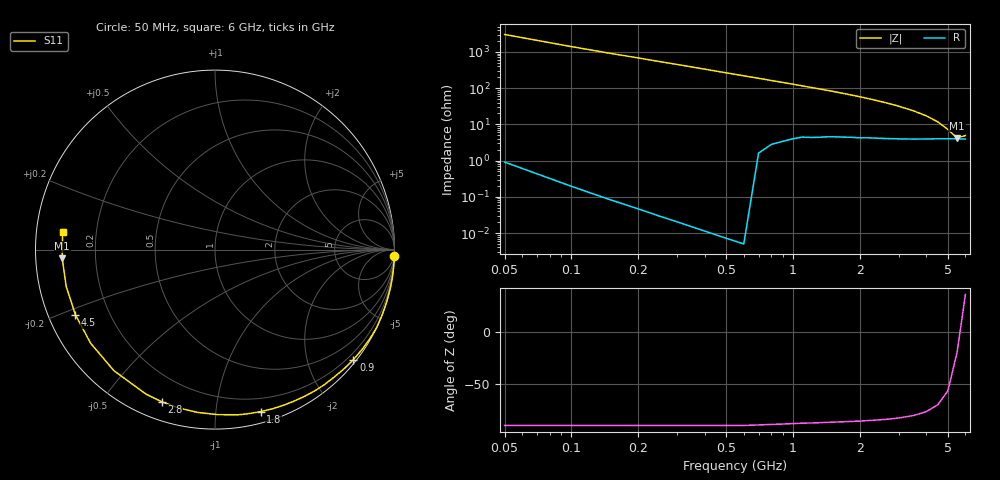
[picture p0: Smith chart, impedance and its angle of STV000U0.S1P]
! SIEMENS Discrete & RF Semiconductors
! BA892
! Si PIN Diode in SCD-80
! VR = 0 V
! S-Parameters:  September  1997
# GHz  S  MA  R  50
!  f  S11
! GHz  MAG  ANG
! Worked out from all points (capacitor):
!   34 points, 50 MHz to 6 GHz, reference 50 ohm
!   read as one part to ground: C = 1.14 pF near 50 MHz
!   lowest |Z| = 4.23 ohm at 5.5 GHz (marker M1)
!   series resonance near 5.665 GHz, so ESL is about 690 pH
!   S11 on the Smith chart (normalised r, x): 50 MHz: 0, -60; 900 MHz: 0.07, -2.86; 1.8 GHz: 0.09, -1.32; 2.8 GHz: 0.08, -0.71; 4.5 GHz: 0.08, -0.22; 6 GHz: 0.08, +0.06
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0.05  1 -1.9
0.2  1 -8.4
0.3  1 -12.7
0.4  1 -17.1
0.5  1 -21.5
0.6  1 -25.8
0.7  0.9957 -30.0
0.8  0.9902 -34.4
0.9  0.9853 -38.5
1  0.979 -42.7
1.1  0.9723 -46.8
1.2  0.9683 -50.9
1.3  0.9635 -54.9
1.4  0.9572 -58.9
1.6  0.947 -66.7
1.8  0.9377 -74.3
2  0.9297 -81.8
2.2  0.9198 -89.0
2.4  0.9122 -96.1
2.6  0.9054 -102.7
2.8  0.8981 -109.3
3  0.8924 -115.5
3.5  0.8788 -129.9
4  0.8674 -143.0
4.5  0.8584 -155.0
5  0.8541 -166.1
5.5  0.8527 -176.7
6  0.8547 173.3
